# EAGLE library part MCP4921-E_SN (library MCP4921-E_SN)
Single 12-bit DAC SPI I/F,MCP4921-E/SN Source: Datasheet
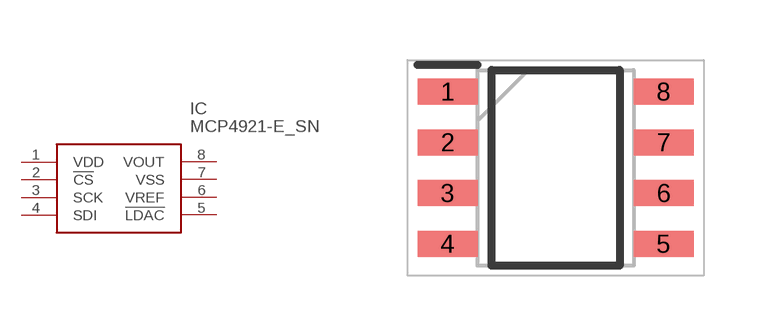
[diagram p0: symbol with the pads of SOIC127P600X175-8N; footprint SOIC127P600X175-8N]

Designator prefix IC

## MCP4921-E_SN (Description: Single 12-bit DAC SPI I/F,MCP4921-E/SN; Height: 1.75mm; Manufacturer_Name: Microchip; Manufacturer_Part_Number: MCP4921-E/SN; Mouser_Part_Number: 579-MCP4921-E/SN; Mouser_Price-Stock: https://www.mouser.co.uk/ProductDetail/Microchip-Technology/MCP4921-E-SN?qs=W2ndVjZwIIIOYoIsyQyMYw%3D%3D)  [SOIC127P600X175-8N]
1  VDD
2  !CS
3  SCK
4  SDI
5  !LDAC
6  VREF
7  VSS
8  VOUT

## Footprint SOIC127P600X175-8N (pad centres in mm)
8 lead soic-
smd 1.5 x 0.65: 1 -2.7,1.905; 2 -2.7,0.635; 3 -2.7,-0.635; 4 -2.7,-1.905; 5 2.7,-1.905; 6 2.7,-0.635; 7 2.7,0.635; 8 2.7,1.905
